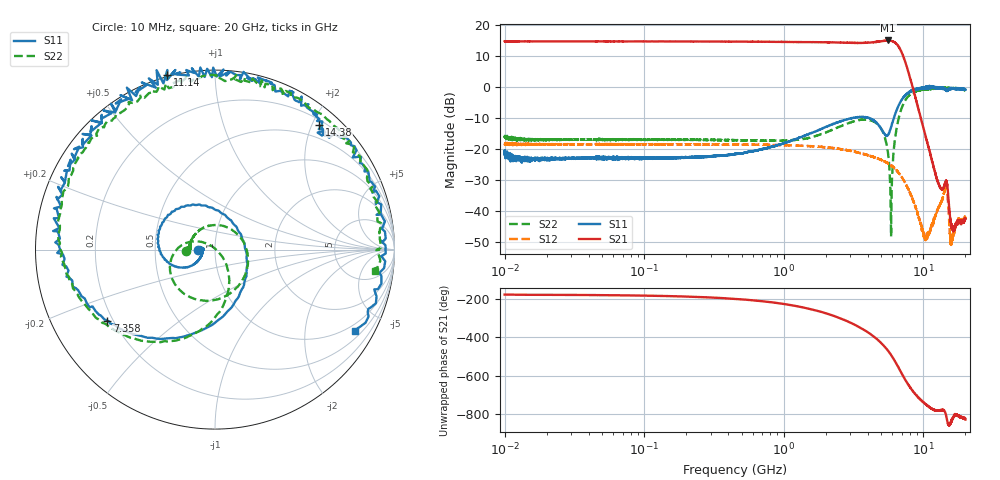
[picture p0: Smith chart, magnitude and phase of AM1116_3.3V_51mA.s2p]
!Agilent Technologies,E8364B,MY43040894,A.07.50.67
!Agilent E8364B: A.07.50.67
!Date: Monday, June 21, 2021 12:17:40
!Correction: S11(Full 2 Port(1,2))
!S21(Full 2 Port(1,2))
!S12(Full 2 Port(1,2))
!S22(Full 2 Port(1,2))
!S2P File: Measurements: S11, S21, S12, S22:Log Frequency Sweep
# Hz S  dB  R 50
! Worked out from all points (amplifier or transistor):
!   6401 points, 10 MHz to 20 GHz, reference 50 ohm
!   highest |S21| = 15.0 dB at 5.592 GHz (marker M1)
!   |S21| within 3 dB of that: start of sweep to 6.841 GHz
!   unconditionally stable (mu >= 1): start of sweep to 9.773 GHz; 9.91 GHz to 10.12 GHz; 12.57 GHz to end of sweep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
!   at 35.47 MHz: K = 1.08, MAG = 14.8 dB, |S12| = -18.4 dB
!   at 447.2 MHz: K = 1.09, MAG = 14.8 dB, |S12| = -18.6 dB
!   at 20 GHz: K = 319.85, MAG = -28.1 dB, |S12| = -42.4 dB
!   S11 on the Smith chart (normalised r, x): 10 MHz: 0.83, -0.01; 7.358 GHz: 0.18, -0.29; 11.14 GHz: -0.01, +0.76; 14.38 GHz: 0.27, +2.11; 20 GHz: 0.73, -3.58
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1e7  -20.53 -177.5  14.73 -179.4  -18.33 -1.5  -15.88 -176.9
3.550942e7  -23.02 -176.9  14.72 178.5  -18.44 -1.9  -16.96 177.0
1.260919e8  -22.84 -170.0  14.71 173.9  -18.45 -5.7  -17.01 168.4
4.472136e8  -21.51 -156.4  14.65 158.5  -18.55 -19.6  -17.11 139.0
9.152377e8  -18.62 -146.6  14.56 135.9  -18.69 -40.1  -17.25 93.6
1.58803e9  -14.76 -147.6  14.49 103.8  -19.09 -69.4  -16.10 26.8
2.538599e9  -11.10 -167.5  14.35 57.9  -19.99 -110.7  -12.68 -50.6
3.091822e9  -10.04 176.1  14.25 30.8  -20.66 -134.5  -11.17 -85.3
3.779047e9  -9.73 151.2  14.26 -3.3  -21.63 -164.3  -10.49 -122.5
4.652055e9  -11.58 108.5  14.58 -50.1  -22.93 158.2  -11.80 -164.7
5.183002e9  -14.58 61.4  14.89 -82.3  -23.84 134.0  -14.97 170.5
5.592316e9  -15.38 -0.7  15.03 -110.9  -24.61 114.4  -21.59 149.6
5.639001e9  -14.92 -7.2  15.01 -114.5  -24.75 112.3  -23.10 146.9
6.041124e9  -11.09 -60.1  14.76 -146.0  -25.69 92.8  -24.19 -45.3
6.372768e9  -7.96 -89.0  14.02 -174.3  -26.70 77.1  -14.33 -65.7
6.859728e9  -4.69 -121.1  11.97 143.4  -28.37 53.9  -7.85 -92.9
7.357635e9  -2.86 -146.3  8.55 104.3  -30.70 31.9  -4.56 -119.5
8.187644e9  -1.28 180.0  1.59 52.2  -35.10 1.7  -2.11 -156.5
1.113647e10  0.10 105.3  -21.15 -44.8  -46.51 25.9  -0.66 125.6
1.437611e10  -0.85 50.1  -30.83 -72.0  -32.72 -54.3  -0.47 71.8
1.599787e10  -0.54 30.9  -45.88 -109.1  -48.90 -86.5  -0.36 48.3
2e10  -0.89 -30.1  -42.53 -106.5  -42.39 -101.8  -0.94 -7.7
